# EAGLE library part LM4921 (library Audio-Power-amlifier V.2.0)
LM4921 Low Voltage I2S 16-Bit Stereo DAC with Stereo Headphone Power Amplifiers and Volume Control
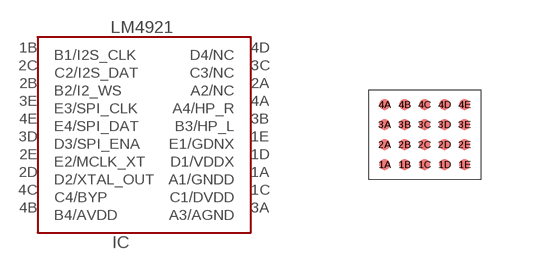
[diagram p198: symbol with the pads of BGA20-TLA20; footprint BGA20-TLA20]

Designator prefix IC

## LM4921  [BGA20-TLA20]
1A  A1/GNDD  pwr
1B  B1/I2S_CLK
1C  C1/DVDD  pwr
1D  D1/VDDX  pwr
1E  E1/GDNX  pwr
2A  A2/NC  nc
2B  B2/I2_WS
2C  C2/I2S_DAT  in
2D  D2/XTAL_OUT  out
2E  E2/MCLK_XT  in
3A  A3/AGND  pwr
3B  B3/HP_L  out
3C  C3/NC  nc
3D  D3/SPI_ENA  in
3E  E3/SPI_CLK  in
4A  A4/HP_R  out
4B  B4/AVDD  pwr
4C  C4/BYP
4D  D4/NC  nc
4E  E4/SPI_DAT  in

## Footprint BGA20-TLA20 (pad centres in mm)
DSBGA20-TLA20_ 2.792x2.258 BODY. www.ti.com/audio
smd 0.275 x 0.275: 1A -1,-0.75; 1B -0.5,-0.75; 1C 0,-0.75; 1D 0.5,-0.75; 1E 1,-0.75; 2A -1,-0.25; 2B -0.5,-0.25; 2C 0,-0.25; 2D 0.5,-0.25; 2E 1,-0.25; 3A -1,0.25; 3B -0.5,0.25; 3C 0,0.25; 3D 0.5,0.25; 3E 1,0.25; 4A -1,0.75; 4B -0.5,0.75; 4C 0,0.75; 4D 0.5,0.75; 4E 1,0.75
